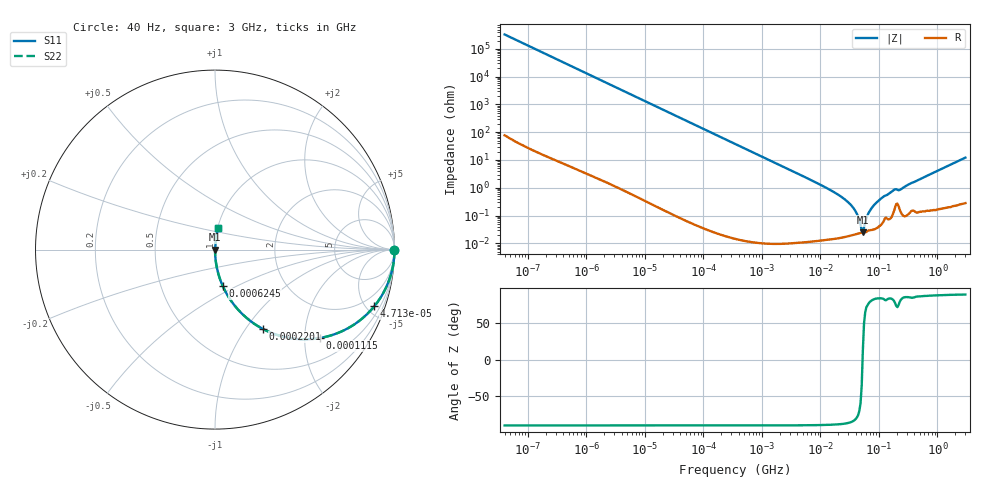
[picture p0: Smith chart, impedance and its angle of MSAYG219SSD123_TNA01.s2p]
! MSAYG219SSD123_TNA01  S-PARAMETER MODEL  ( General Type )
! Model Generated by TAIYO YUDEN Corporation (http://www.ty-top.com)
! Version 2.0
! TAIYO YUDEN Control No. 031016
! Copyright(c) 2003 TAIYO YUDEN CO.,LTD. All Rights Reserved.
! Product Description (link to TY-COMPAS)
! https://ds.yuden.co.jp/TYCOMPAS/or/detail?pn=MSAYG219SSD123KTNA01&u=M
! Products Name : Multilayer Ceramic Capacitors
! Characteristics :
!  Capacitance : 0.012 uF , Rated Voltage : 35V
!  Case Size : 2.0 x 1.25 / 0.079 x 0.049 [mm/inch] , Thickness : 0.85 / 0.033 [mm/inch]
!  (Conditions: Temperature = 25 degC , DC Bias Current/Voltage = 0A / 0V)
! External Node Assignments :
!  1  o---| |---o  2
! GND o---------o GND
! Frequency Range : 40Hz  -  3GHz  [ 401 STEP ]
# MHz S RI R 50
! Freq[MHz].  S11 Real  S11 Imag  S21 Real  S21 Imag  S12 Real  S12 Imag  S22 Real  S22 Imag
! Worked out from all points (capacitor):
!   401 points, 40 Hz to 3 GHz, reference 50 ohm
!   read as one part in series: C = 12 nF near 44 Hz
!   lowest |Z| = 25.2 mohm at 53.08 MHz (marker M1)
!   series resonance near 52.5 MHz, so ESL is about 770 pH
!   S11 on the Smith chart (normalised r, x): 40 Hz: open; 47.13 kHz: 1.00, -5.63; 111.5 kHz: 1.00, -2.38; 220.1 kHz: 1.00, -1.21; 624.5 kHz: 1.00, -0.42; 3 GHz: 1.01, +0.24
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4e-05  1 -0.000302  1.61e-07 0.000302  1.61e-07 0.000302  1 -0.000302
0.000834  1 -0.00629  4.1e-05 0.00629  4.1e-05 0.00629  1 -0.00629
0.017386  0.9831 -0.1288  0.0169 0.1288  0.0169 0.1288  0.9831 -0.1288
0.047134  0.8878 -0.3154  0.1122 0.3154  0.1122 0.3154  0.8878 -0.3154
0.111532  0.5858 -0.4924  0.4142 0.4924  0.4142 0.4924  0.5858 -0.4924
0.220148  0.2664 -0.4419  0.7336 0.4419  0.7336 0.4419  0.2664 -0.4419
0.362475  0.1182 -0.3226  0.8818 0.3226  0.8818 0.3226  0.1182 -0.3226
0.624497  0.0433 -0.2032  0.9567 0.2032  0.9567 0.2032  0.0433 -0.2032
1.693006  0.00618 -0.0778  0.9938 0.0778  0.9938 0.0778  0.00618 -0.0778
7.222098  0.00044 -0.018  0.9996 0.018  0.9996 0.018  0.00044 -0.018
17.08948  0.000191 -0.00692  0.9998 0.00692  0.9998 0.00692  0.000191 -0.00692
29.4429  0.000187 -0.00306  0.9998 0.00306  0.9998 0.00306  0.000187 -0.00306
38.64618  0.00021 -0.00156  0.9998 0.00156  0.9998 0.00156  0.00021 -0.00156
42.31378  0.00022 -0.00108  0.9998 0.00108  0.9998 0.00108  0.00022 -0.00108
48.47801  0.000236 -0.000395  0.9998 0.000395  0.9998 0.000395  0.000236 -0.000395
53.07868  0.000245 5.64e-05  0.9998 -5.64e-05  0.9998 -5.64e-05  0.000245 5.64e-05
55.54024  0.000249 0.000289  0.9998 -0.000289  0.9998 -0.000289  0.000249 0.000289
66.58224  0.00029 0.00121  0.9997 -0.00121  0.9997 -0.00121  0.00029 0.00121
79.8195  0.000318 0.00218  0.9997 -0.00218  0.9997 -0.00218  0.000318 0.00218
109.6283  0.000482 0.00412  0.9995 -0.00412  0.9995 -0.00412  0.000482 0.00412
150.5692  0.000772 0.00623  0.9992 -0.00623  0.9992 -0.00623  0.000772 0.00623
3000  0.0172 0.1191  0.9828 -0.1191  0.9828 -0.1191  0.0172 0.1191
